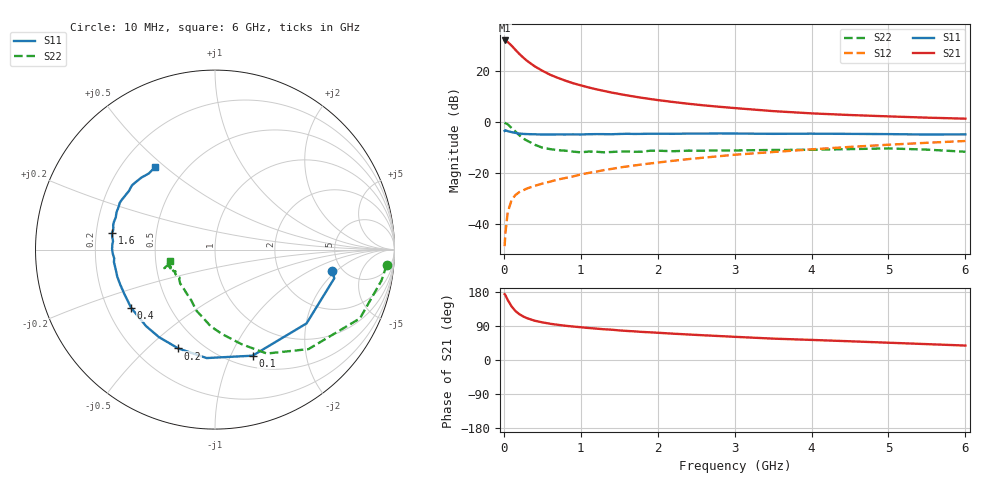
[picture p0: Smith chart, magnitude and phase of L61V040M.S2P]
!  INFINEON TECHNOLOGIES Small Signal Semiconductors
! BFR380L3 , Si-NPN RF-Transistor in TSLP-3-1
!  Vce=1 V,  Ic=40 mA
! Common Emitter S-Parameters:  07. March 2005
#  GHz  S  MA  R  50
! f  S11  S21  S12  S22
! GHz  Mag  Ang  Mag  Ang  Mag  Ang  Mag  Ang
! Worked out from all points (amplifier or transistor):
!   36 points, 10 MHz to 6 GHz, reference 50 ohm
!   highest |S21| = 32.0 dB at 10 MHz (marker M1)
!   |S21| within 3 dB of that: start of sweep to 129.8 MHz
!   unconditionally stable (mu >= 1): 1.526 GHz to 5.579 GHz
!   at 250 MHz: K = 0.46, MSG = 26.1 dB, |S12| = -26.9 dB
!   at 1.4 GHz: K = 1.00, MSG = 15.0 dB, |S12| = -18.5 dB
!   at 6 GHz: K = 0.99, MSG = 4.4 dB, |S12| = -7.5 dB
!   S11 on the Smith chart (normalised r, x): 10 MHz: 4.14, -1.79; 100 MHz: 0.62, -1.21; 200 MHz: 0.37, -0.63; 400 MHz: 0.30, -0.29; 1.6 GHz: 0.27, +0.07; 6 GHz: 0.34, +0.46
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0.01  0.664 -10.5  39.71 173.8  0.0036 79.2  0.9602 -5.1
0.02  0.6836 -13.5  39.16 171.4  0.0064 82.2  0.9431 -10.6
0.05  0.6552 -38.9  37.11 158.6  0.0165 75.6  0.8938 -25.4
0.1  0.627 -70.5  31.49 141.7  0.029 61.7  0.7607 -46.8
0.15  0.6061 -94.4  26.04 129.4  0.0364 54.1  0.647 -63.5
0.2  0.5874 -110.4  21.7 121.1  0.0414 51.7  0.5475 -74.3
0.25  0.5789 -122.7  18.43 115.1  0.045 49.6  0.4716 -85.3
0.3  0.5739 -131.9  15.85 110.4  0.0489 49.1  0.4283 -93.1
0.4  0.5689 -145.2  12.36 103.7  0.0551 49.8  0.3551 -107.0
0.5  0.5624 -153.8  10.1 99.3  0.0611 51.2  0.3113 -115.3
0.6  0.563 -159.9  8.448 95.7  0.0666 53.6  0.2911 -122.8
0.7  0.565 -164.5  7.321 92.9  0.0733 55.3  0.277 -129.7
0.9  0.5673 -173.0  5.733 88.3  0.0845 58.2  0.2597 -140.1
1.1  0.5706 -178.0  4.746 84.5  0.0988 60.2  0.26 -144.7
1.3  0.5725 176.8  4.051 81.1  0.1124 61.3  0.2516 -151.6
1.6  0.5818 170.9  3.309 76.7  0.1325 62.6  0.2614 -156.5
2.2  0.5812 162.0  2.452 69.5  0.1716 63.2  0.2645 -158.3
2.8  0.5911 153.8  1.976 63.2  0.211 63.3  0.2735 -162.4
3.5  0.5803 145.6  1.623 56.4  0.2551 61.1  0.28 -161.4
4.5  0.5795 139.3  1.36 49.4  0.3214 59.0  0.2908 -160.7
5.5  0.5623 131.1  1.208 41.9  0.3872 54.8  0.2841 -161.4
6  0.5674 126.1  1.153 38.1  0.4201 52.4  0.2581 -165.8
